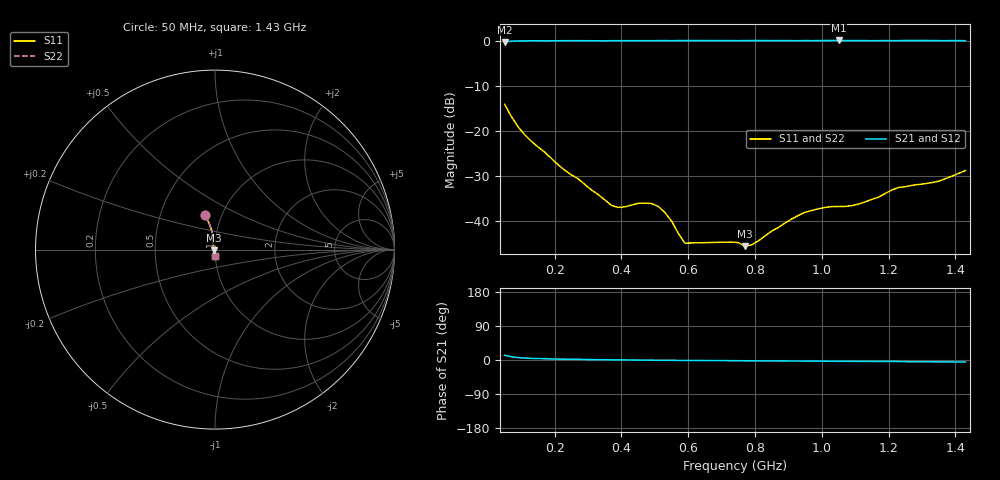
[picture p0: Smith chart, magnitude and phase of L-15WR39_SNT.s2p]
! P/N: L-15WR39JV4
! Measured by Marlon B.  (Application Engineer Tech)
! Measured on Oct. 14, 2004
! Measured with 8720C VNA with Shunt-Through Fixture, TRL* calibration used
#	mhz	s	ma	r	50
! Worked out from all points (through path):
!   64 points, 50 MHz to 1.43 GHz, reference 50 ohm
!   highest |S21| = 0.07 dB at 1.05 GHz (marker M1); lowest = -0.3 dB at 50 MHz (marker M2)
!   group delay of S21, straight-line fit = 20.7 ps
!   lowest |S11| = -45.5 dB at 770 MHz (marker M3), VSWR 1.01, Z = 49.6 - j0.325 ohm
!   |S11| at or under -10 dB: start of sweep to end of sweep
!   |S22| runs from -45.5 to -14.1 dB; largest |S21 - S12| = 0
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50  0.198 106.0  0.9715 12.5  0.9715 12.5  0.198 106.0
90  0.1117 100.0  0.9959 6.4  0.9959 6.4  0.1117 100.0
110  0.09091 99.6  0.9983 5.1  0.9983 5.1  0.09091 99.6
210  0.04231 106.6  1.001 2.3  1.001 2.3  0.04231 106.6
290  0.0256 106.1  1.001 1.5  1.001 1.5  0.0256 106.1
370  0.01499 101.5  1.002 0.5  1.002 0.5  0.01499 101.5
390  0.01424 96.8  1.003 0.3  1.003 0.3  0.01424 96.8
470  0.01592 111.4  1.003 -0.3  1.003 -0.3  0.01592 111.4
510  0.01461 132.7  1.004 -0.8  1.004 -0.8  0.01461 132.7
550  0.01006 155.3  1.003 -0.9  1.003 -0.9  0.01006 155.3
590  0.00573 163.6  1.006 -1.1  1.006 -1.1  0.00573 163.6
750  0.0058 -145.0  1.002 -1.9  1.002 -1.9  0.0058 -145.0
770  0.0053 -141.7  1.005 -2.0  1.005 -2.0  0.0053 -141.7
790  0.00548 -139.8  1.006 -2.1  1.006 -2.1  0.00548 -139.8
910  0.01061 -126.7  1.003 -2.7  1.003 -2.7  0.01061 -126.7
970  0.01317 -115.2  1.003 -2.9  1.003 -2.9  0.01317 -115.2
1050  0.01458 -103.2  1.008 -3.5  1.008 -3.5  0.01458 -103.2
1110  0.01552 -101.9  1.005 -3.7  1.005 -3.7  0.01552 -101.9
1170  0.01851 -104.9  1.004 -4.0  1.004 -4.0  0.01851 -104.9
1210  0.02225 -102.9  1.003 -3.8  1.003 -3.8  0.02225 -102.9
1350  0.02776 -97.7  1.004 -4.9  1.004 -4.9  0.02776 -97.7
1430  0.03644 -94.1  1.002 -5.3  1.002 -5.3  0.03644 -94.1
